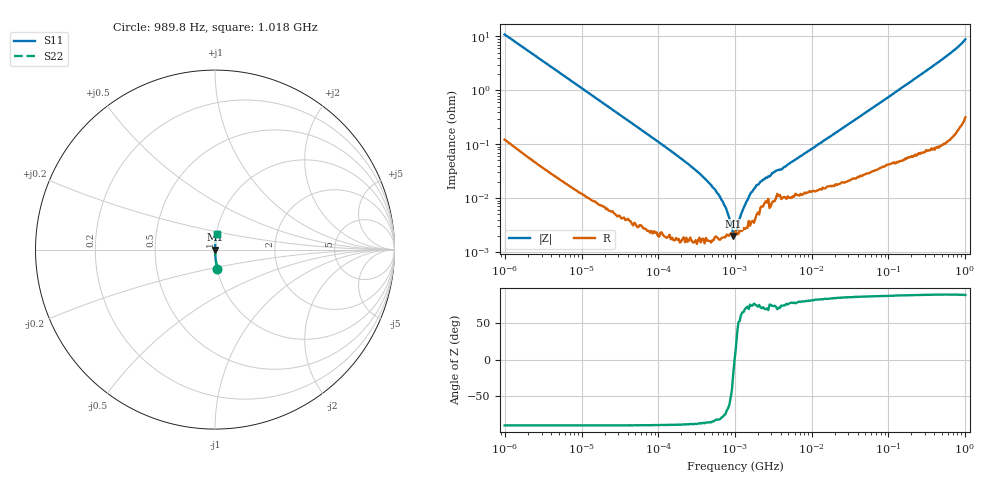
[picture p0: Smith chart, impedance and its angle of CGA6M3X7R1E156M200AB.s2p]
! S-Parameter Data Generated by TDK Corporation
! Copyright(C) 2024 TDK Corporation.
! All Rights Reserved.
! TDK P/N: CGA6M3X7R1E156M200AB (Multilayer Ceramic Chip Capacitor)
! Property: C=15uF
! Size(LxWxT): 3.2x2.5x2mm
! Model Type: s2p (Touchstone File Format Version 1.0)
! Frequency: DC=Yes Start=0.000989846MHz Stop=1017.91MHz 409points Log-sweep
! Model Generated on May 28, 2024
! Terms and conditions regarding TDK Simulation Models:
! 1)This simulation model is being provided solely for informational
!  purposes. Please refer to the specifications of the products in
!  terms of detailed characteristics of such products.
! 2)In no event shall TDK Corporation of any of its subsidiaries be
!  liable for any loss or damage arising, directly or indirectly,
!  from any information contained in this simulation model, including,
!  but not limited to loss or damages arising from any inaccuracies,
!  omissions or errors in connection with such information.
! 3)Any and all copyrights on this simulation model are owned by
!  TDK Corporation.  Duplication or redistribution of this simulation
!  model without prior written permission from TDK Corporation
!  is prohibited.
! 4)This simulation model is subject to any modification or change
!  without any prior notice.
! 5)Neither TDK Corporation nor any of its subsidiaries shall make any
!  warranty, express or implied, including but not limited to the
!  correctness, implied warranties of merchantability and fitness for
!  a particular purpose with respect to this simulation models.
! 6)The use of this simulation model shall be deemed to have consented
!  to the terms and conditions hereof.
! Port Assignments:
!  1 ---| |--- 2
! Applicable Conditions:
!  Temperature = 25 degC
!  DC Bias Voltage = 0 V
!  Small Signal Operation
# Hz S MA R 50
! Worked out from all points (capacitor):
!   408 points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, 989.8 Hz to 1.018 GHz, reference 50 ohm
!   read as one part in series: C = 14.7 uF near 1.07 kHz
!   lowest |Z| = 1.98 mohm at 950.5 kHz (marker M1)
!   series resonance near 991.6 kHz, so ESL is about 1.8 nH
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989.846  0.1082 -83.1  0.9929 6.2  0.9929 6.2  0.1082 -83.1
2625.44  0.04152 -87.0  0.9987 2.4  0.9987 2.4  0.04152 -87.0
10287  0.01072 -88.8  0.9998 0.6  0.9998 0.6  0.01072 -88.8
102818  0.001077 -88.9  1 0.1  1 0.1  0.001077 -88.9
233303  0.0004563 -87.7  1 0.0  1 0.0  0.0004563 -87.7
331458  0.0003013 -86.8  1 0.0  1 0.0  0.0003013 -86.8
452889  0.0001961 -85.3  1 0.0  1 0.0  0.0001961 -85.3
643429  0.0001036 -80.6  1 0.0  1 0.0  0.0001036 -80.6
695651  8.588e-05 -77.5  1 0.0  1 0.0  8.588e-05 -77.5
950505  1.979e-05 -20.0  1 0.0  1 0.0  1.979e-05 -20.0
1027650  2.51e-05 14.3  1 -0.0  1 -0.0  2.51e-05 14.3
1350400  7.366e-05 68.7  1 -0.0  1 -0.0  7.366e-05 68.7
1460000  9.206e-05 72.2  1 -0.0  1 -0.0  9.206e-05 72.2
1994880  0.0001764 72.2  0.9999 -0.0  0.9999 -0.0  0.0001764 72.2
2331840  0.0002205 71.5  0.9999 -0.0  0.9999 -0.0  0.0002205 71.5
3312890  0.0003081 73.3  0.9999 -0.0  0.9999 -0.0  0.0003081 73.3
4353360  0.000374 73.7  0.9999 -0.0  0.9999 -0.0  0.000374 73.7
1.02712e7  0.000833 80.6  0.9999 -0.0  0.9999 -0.0  0.000833 80.6
1.0266e8  0.007633 86.4  0.9996 -0.4  0.9996 -0.4  0.007633 86.4
5.58375e8  0.04156 86.2  0.9981 -2.4  0.9981 -2.4  0.04156 86.2
7.847e8  0.06087 84.9  0.9965 -3.5  0.9965 -3.5  0.06087 84.9
1.01791e9  0.08823 82.9  0.993 -5.1  0.993 -5.1  0.08823 82.9
